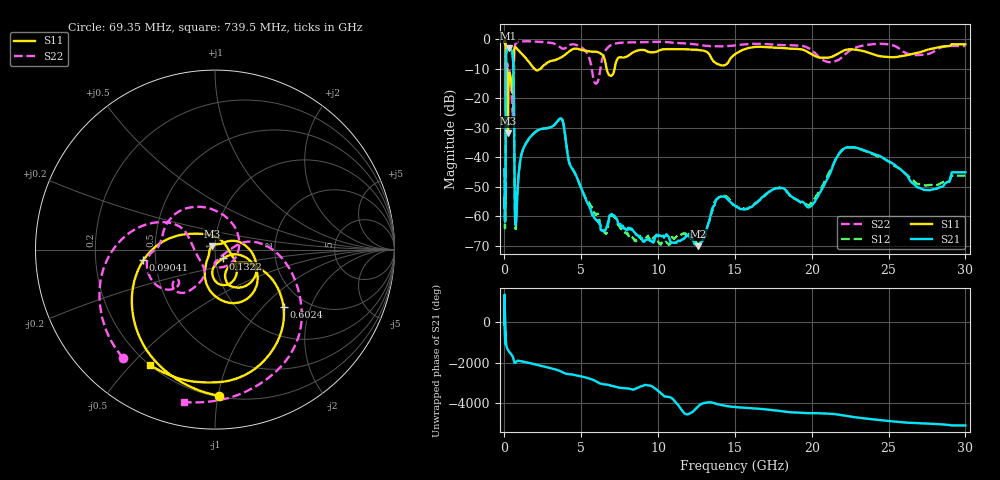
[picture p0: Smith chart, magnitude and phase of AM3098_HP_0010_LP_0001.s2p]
! Date/Time: Thu, Feb 28, 2019 8:32 AM
! Network Analyzer: Agilent Technologies E8364B Rev: A.07.50.67
! Sweep from 0.010 to 30.000 GHz, 1601 Points, Sweep Type: LOG
! Power Supply: 5.023 V, 0.002 A
# Hz S DB R 50
!freq MagS11 AngS11 MagS21 AngS21 MagS12 AngS12 MagS22 AngS22
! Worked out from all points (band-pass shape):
!   1601 points, 10 MHz to 30 GHz, reference 50 ohm
!   highest |S21| = -2.99 dB at 265.1 MHz (marker M1); lowest = -70.1 dB at 12.62 GHz (marker M2)
!   |S21| within 3 dB of the highest: 106.3 MHz to 546.3 MHz (440 MHz wide, 135 % of centre)
!   lowest |S11| = -31.8 dB at 228.2 MHz (marker M3), VSWR 1.05, Z = 48.5 + j2.03 ohm
!   |S11| at or under -10 dB: 175.6 MHz to 571.1 MHz (395.5 MHz wide, 106 % of centre); 1.965 GHz to 2.332 GHz (367.2 MHz wide, 17.1 % of centre); 6.649 GHz to 7.166 GHz (517 MHz wide, 7.49 % of centre)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
!   |S22| runs from -25.9 to -0.5 dB; largest |S21 - S12| = 0.01
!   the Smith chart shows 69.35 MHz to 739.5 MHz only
!   S11 on the Smith chart (normalised r, x): 69.35 MHz: 0.21, -1.00; 90.41 MHz: 0.43, -0.06; 132.2 MHz: 1.09, -0.11; 602.4 MHz: 1.55, -1.32; 739.5 MHz: 0.20, -0.57
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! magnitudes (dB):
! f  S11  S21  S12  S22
! 10 MHz  -0.3  -44.0  -44.0  -0.5
! 38.04 MHz  -0.5  -60.6  -60.9  -0.8
! 69.35 MHz  -1.8  -51.6  -53.8  -2.0
! 90.41 MHz  -7.9  -19.5  -19.5  -9.4
! 132.2 MHz  -23.5  -3.9  -3.9  -11.5
! 144.7 MHz  -13.9  -3.6  -3.5  -10.3
! 186.8 MHz  -11.5  -3.4  -3.4  -8.2
! 228.2 MHz  -31.8  -3.1  -3.0  -9.9
! 265.1 MHz  -15.2  -3.0  -3.0  -10.4
! 550.5 MHz  -13.5  -6.3  -6.2  -25.9
! 602.4 MHz  -6.0  -14.4  -14.4  -12.3
! 679.2 MHz  -2.6  -58.5  -56.8  -2.2
! 739.5 MHz  -2.6  -61.6  -64.2  -1.2
! 1.044 GHz  -4.4  -40.6  -40.5  -0.7
! 2.084 GHz  -10.5  -31.2  -31.0  -0.7
! 3.704 GHz  -6.0  -26.8  -26.8  -2.9
! 5.959 GHz  -4.2  -61.2  -59.6  -15.0
! 7.926 GHz  -5.9  -64.5  -65.6  -1.0
! 12.62 GHz  -3.6  -70.1  -69.4  -1.8
! 19.9 GHz  -4.7  -56.7  -55.9  -3.2
! 22.56 GHz  -3.4  -36.5  -36.7  -3.5
! 30 GHz  -1.6  -45.1  -46.2  -2.2
